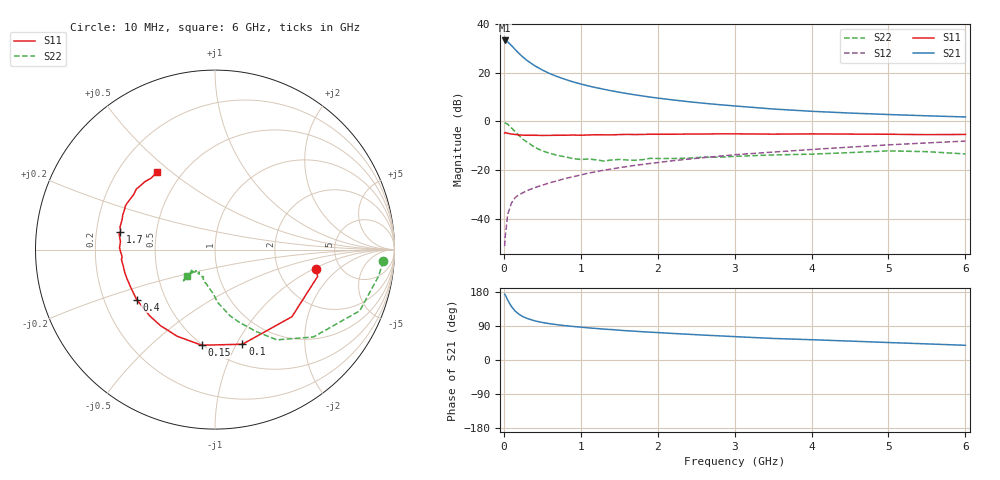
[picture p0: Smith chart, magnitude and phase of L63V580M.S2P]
!  INFINEON TECHNOLOGIES Small Signal Semiconductors
! BFR380L3 , Si-NPN RF-Transistor in TSLP-3-1
!  Vce=3.5 V,  Ic=80 mA
! Common Emitter S-Parameters:  07. March 2005
#  GHz  S  MA  R  50
! f  S11  S21  S12  S22
! GHz  Mag  Ang  Mag  Ang  Mag  Ang  Mag  Ang
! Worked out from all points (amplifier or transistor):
!   36 points, 10 MHz to 6 GHz, reference 50 ohm
!   highest |S21| = 33.3 dB at 10 MHz (marker M1)
!   |S21| within 3 dB of that: start of sweep to 126.2 MHz
!   unconditionally stable (mu >= 1): 1.193 GHz to 4.845 GHz
!   at 250 MHz: K = 0.55, MSG = 27.9 dB, |S12| = -29.3 dB
!   at 1.4 GHz: K = 1.02, MAG = 15.2 dB, |S12| = -19.6 dB
!   at 6 GHz: K = 0.97, MSG = 5.0 dB, |S12| = -8.1 dB
!   S11 on the Smith chart (normalised r, x): 10 MHz: 3.30, -1.07; 100 MHz: 0.70, -1.06; 150 MHz: 0.49, -0.74; 400 MHz: 0.34, -0.26; 1.7 GHz: 0.30, +0.09; 6 GHz: 0.37, +0.45
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0.01  0.5722 -11.0  46.4 173.8  0.0027 75.2  0.9395 -3.9
0.02  0.5912 -14.6  46.06 171.2  0.0045 82.3  0.9239 -9.1
0.05  0.5688 -41.1  43.28 158.0  0.0122 74.0  0.8757 -22.9
0.1  0.549 -73.8  36.42 140.8  0.0211 64.4  0.7332 -41.6
0.15  0.5379 -97.9  29.91 128.5  0.0273 57.0  0.6094 -55.6
0.2  0.5269 -113.6  24.79 120.3  0.0311 56.6  0.5087 -63.5
0.25  0.5212 -125.8  21.02 114.4  0.0341 54.4  0.4254 -71.7
0.3  0.5182 -134.5  18.03 109.8  0.0375 54.9  0.3777 -77.3
0.4  0.5179 -147.5  14.05 103.4  0.0432 56.5  0.2947 -87.1
0.5  0.5145 -155.6  11.45 99.1  0.0486 58.8  0.2474 -92.0
0.6  0.5162 -161.4  9.594 95.6  0.0548 60.1  0.2204 -97.7
0.7  0.5186 -165.5  8.306 93.0  0.0602 62.2  0.1987 -103.6
0.9  0.5241 -173.9  6.504 88.5  0.0726 64.7  0.1714 -113.0
1.1  0.5259 -178.6  5.375 84.8  0.0862 66.3  0.1685 -117.9
1.4  0.5287 175.0  4.262 80.3  0.1047 67.4  0.1607 -123.9
1.7  0.5362 169.3  3.531 76.0  0.1242 68.0  0.1581 -132.0
2.2  0.5442 161.9  2.764 70.0  0.1552 68.0  0.1723 -133.0
2.8  0.5551 154.0  2.211 63.7  0.1921 67.7  0.1834 -138.6
3.5  0.547 145.9  1.8 56.9  0.2336 65.4  0.2041 -136.7
4.5  0.5479 139.8  1.486 49.9  0.296 63.5  0.2279 -135.9
5.5  0.5339 131.7  1.304 42.5  0.3607 59.5  0.2383 -135.6
6  0.5391 126.7  1.235 38.8  0.3937 57.3  0.2139 -137.5
